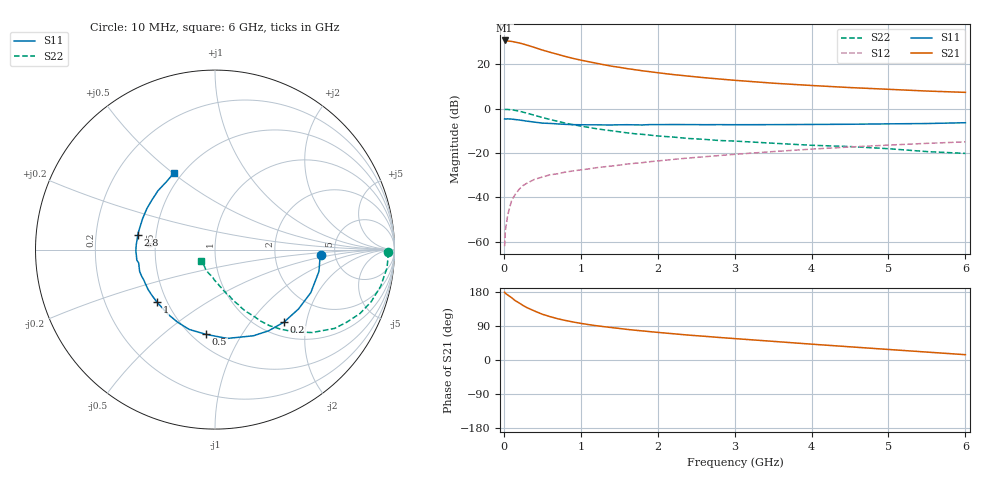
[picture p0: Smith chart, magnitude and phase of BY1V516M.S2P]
! SIEMENS Small Signal Semiconductors
! BFY420
! Si NPN RF SIEGET Grounded Emitter Transistor in MICRO-X
! VCE = 1.5 V  IC = 16 mA
! Common Emitter S-Parameters:  October  1996
# GHz  S  MA  R  50
!  f  S11  S21  S12  S22
! GHz  MAG  ANG  MAG  ANG  MAG  ANG  MAG  ANG
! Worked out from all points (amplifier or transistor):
!   36 points, 10 MHz to 6 GHz, reference 50 ohm
!   highest |S21| = 30.8 dB at 10 MHz (marker M1)
!   |S21| within 3 dB of that: start of sweep to 385 MHz
!   unconditionally stable (mu >= 1): 2.073 GHz to end of sweep
!   at 250 MHz: K = 0.27, MSG = 31.9 dB, |S12| = -34.6 dB
!   at 1.4 GHz: K = 0.88, MSG = 22.5 dB, |S12| = -25.8 dB
!   at 6 GHz: K = 1.09, MAG = 9.4 dB, |S12| = -14.9 dB
!   S11 on the Smith chart (normalised r, x): 10 MHz: 3.85, -0.38; 200 MHz: 1.27, -1.49; 500 MHz: 0.58, -0.71; 1 GHz: 0.44, -0.32; 2.8 GHz: 0.39, +0.08; 6 GHz: 0.45, +0.50
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0.01  0.5914 -3.1  34.61 178.9  0.0008 96.7  0.9629 -0.9
0.02  0.5869 -5.3  34.51 176.0  0.0018 88.5  0.9655 -2.1
0.1  0.5852 -24.2  33 164.6  0.0085 81.8  0.9452 -12.5
0.15  0.5709 -35.4  31.66 156.4  0.0119 74.9  0.9171 -18.5
0.2  0.5577 -46.4  30.42 150.5  0.0154 72.8  0.8828 -23.8
0.25  0.542 -56.6  28.86 143.8  0.0186 66.0  0.8377 -28.9
0.3  0.5256 -66.0  27.2 138.2  0.021 65.3  0.7977 -33.4
0.4  0.4996 -82.1  24.06 129.2  0.0257 60.0  0.7114 -40.5
0.5  0.475 -96.1  21.07 120.8  0.0289 57.3  0.6357 -46.1
0.6  0.4674 -107.9  18.78 114.5  0.0324 55.5  0.5732 -50.6
0.7  0.4551 -117.2  16.84 108.9  0.0343 54.7  0.5207 -54.4
0.8  0.4455 -125.6  15.05 104.3  0.0374 52.4  0.4745 -57.3
1  0.4362 -138.0  12.47 96.7  0.0419 53.2  0.4073 -61.5
1.1  0.4341 -144.5  11.51 93.5  0.0441 53.2  0.3806 -63.8
1.4  0.4315 -157.2  9.12 85.6  0.0511 53.1  0.3193 -68.4
1.6  0.4372 -163.7  8.04 80.8  0.0567 52.7  0.2867 -71.4
2.2  0.4411 -179.1  5.897 69.3  0.0721 51.6  0.2303 -78.6
2.8  0.4385 169.0  4.684 59.5  0.0882 48.9  0.1924 -85.0
3.5  0.4385 157.1  3.771 49.2  0.1083 44.9  0.1672 -91.7
4.5  0.4474 141.6  3.002 34.8  0.1375 37.0  0.1406 -102.3
5.5  0.4646 125.8  2.506 20.9  0.1661 28.0  0.1083 -123.8
6  0.4845 118.2  2.341 14.0  0.1794 23.1  0.0985 -139.8
